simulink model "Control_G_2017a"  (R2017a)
settings: Solver=ode113  StartTime=0  StopTime=80  FixedStep=0.01  MaxStep=0.001  RelTol=1e-3  AbsTol=1e-5
undefined symbols (not defined in the file or in its folder): lower_limit, upper_limit, X0

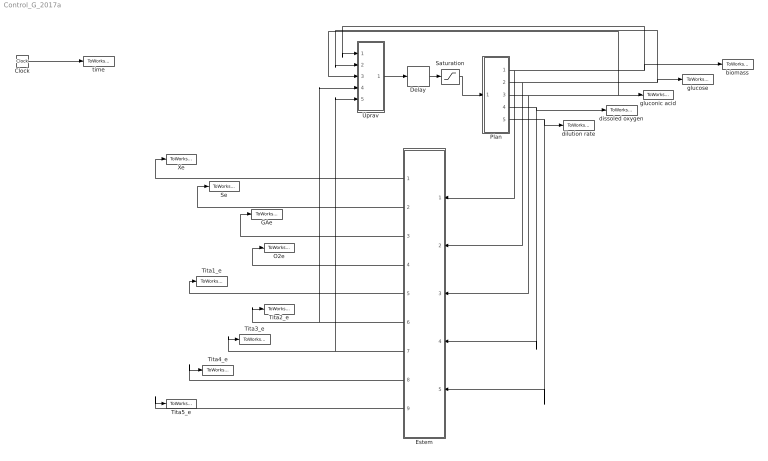
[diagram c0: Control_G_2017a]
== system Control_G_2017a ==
  Clock : Clock
  Delay : TransportDelay  DelayTime=0.0001
  Estem : Subsystem
  GAe : ToWorkspace  VariableName=GAe  SampleTime=0.1
  O2e : ToWorkspace  VariableName=O2e  SampleTime=0.1
  Plan : Subsystem
  Saturation : Saturate  UpperLimit=1  LowerLimit=0.0001
  Se : ToWorkspace  VariableName=Ge  SampleTime=0.1
  Tita1_e : ToWorkspace  VariableName=Tita1_e  SampleTime=0.1
  Tita2_e : ToWorkspace  VariableName=Tita2_e  SampleTime=0.1
  Tita3_e : ToWorkspace  VariableName=Tita3_e  SampleTime=0.1
  Tita4_e : ToWorkspace  VariableName=Tita4_e  SampleTime=0.1
  Tita5_e : ToWorkspace  VariableName=Tita5_e  SampleTime=0.1
  Uprav : Subsystem
  Xe : ToWorkspace  VariableName=Xe  SampleTime=0.1
  biomass : ToWorkspace  VariableName=Xm  SampleTime=0.1
  dilution rate : ToWorkspace  VariableName=D  SampleTime=0.1
  dissoled oxygen : ToWorkspace  VariableName=O2m  SampleTime=0.1
  gluconic acid : ToWorkspace  VariableName=GAm  SampleTime=0.1
  glucose : ToWorkspace  VariableName=Gm  SampleTime=0.1
  time : ToWorkspace  VariableName=time  SampleTime=0.1
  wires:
  Delay/1 -> Saturation/1
  Plan/1(X) -> Estem/1(X), Uprav/1(Xe), biomass/1
  Plan/2(S) -> Uprav/2(Se), glucose/1, Estem/2(S)
  Plan/3(GA) -> Uprav/3(GAe), gluconic acid/1, Estem/3(GA)
  Plan/5(D) -> Estem/5(Din), dilution rate/1
  Uprav/1(D_) -> Delay/1
  Saturation/1 -> Plan/1(D1)
  Plan/4(O2) -> Estem/4(O2), dissoled oxygen/1
  Estem/1(Xe) -> Xe/1
  Estem/2(Se) -> Se/1
  Estem/4(O2e) -> O2e/1
  Estem/5(Tita_1) -> Tita1_e/1
  Estem/7(Tita_3) -> Tita3_e/1, Uprav/5(tita_3)
  Estem/3(GAe) -> GAe/1
  Estem/8(Tita_4) -> Tita4_e/1
  Estem/9(Tita_5) -> Tita5_e/1
  Estem/6(Tita_2) -> Tita2_e/1, Uprav/4(tita_2)
  Clock/1 -> time/1

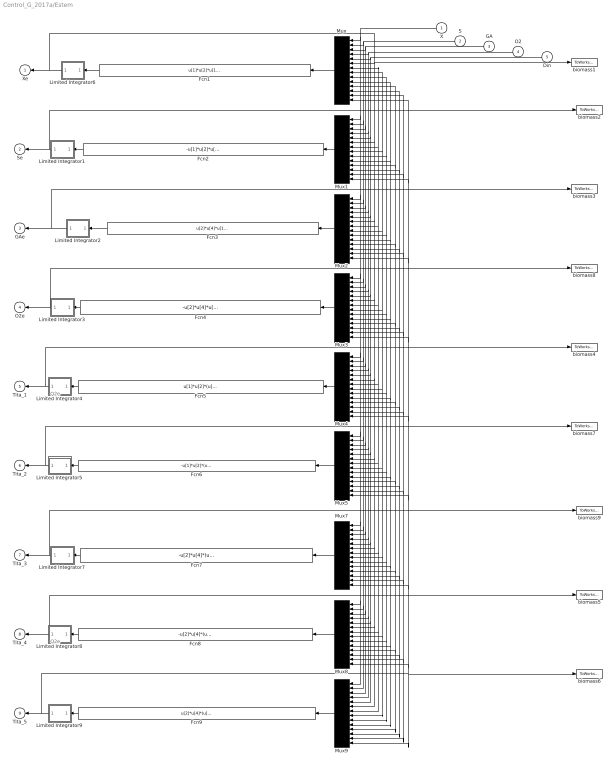
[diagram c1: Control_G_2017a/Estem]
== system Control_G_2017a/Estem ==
  note: Q2e
  note: Q2e
  X : Inport
  S : Inport  Port=2
  GA : Inport  Port=3
  O2 : Inport  Port=4
  Din : Inport  Port=5
  Fcn1 : Fcn  Expr=u[1]*u[2]*u[10]-u[5]*u[1]+1*(u[1]-u[6])
  Fcn2 : Fcn  Expr=-u[1]*u[2]*u[11]-u[2]*u[4]*u[12]-u[5]*(u[2]-200)+1*(u[2]-u[7])
  Fcn3 : Fcn  Expr=u[2]*u[4]*u[14]-u[5]*u[3]+1*(u[3]-u[8])
  Fcn4 : Fcn  Expr=-u[2]*u[4]*u[13]-u[5]*u[4]+600*(0.0075- u[4])+1*(u[4]-u[9])
  Fcn5 : Fcn  Expr=u[1]*u[2]*(u[1]-u[6])/(4*(u[1]*u[2]*u[1]*u[2]))
  Fcn6 : Fcn  Expr=-u[1]*u[2]*(u[2]-u[7])/(4*(u[1]*u[2]*u[1]*u[2]+u[2]*u[4]*u[2]*u[4]))
  Fcn7 : Fcn  Expr=-u[2]*u[4]*(u[2]-u[7])/(4*(u[1]*u[2]*u[1]*u[2]+u[2]*u[4]*u[2]*u[4]))
  Fcn8 : Fcn  Expr=-u[2]*u[4]*(u[4]-u[9])/(4*u[2]*u[4]*u[2]*u[4])
  Fcn9 : Fcn  Expr=u[2]*u[4]*(u[3]-u[8])/(4*u[2]*u[4]*u[2]*u[4])
  Limited Integrator1 : Subsystem
  Limited Integrator2 : Subsystem
  Limited Integrator3 : Subsystem
  Limited Integrator4 : Subsystem
  Limited Integrator5 : Subsystem
  Limited Integrator6 : Subsystem
  Limited Integrator7 : Subsystem
  Limited Integrator8 : Subsystem
  Limited Integrator9 : Subsystem
  Mux{,1..5,7..9} (9 alike) : Mux  Inputs=14
  biomass1 : ToWorkspace  VariableName=Xest  SampleTime=0.1
  biomass2 : ToWorkspace  VariableName=Sest  SampleTime=0.1
  biomass3 : ToWorkspace  VariableName=GAest  SampleTime=0.1
  biomass4 : ToWorkspace  VariableName=Tita1  SampleTime=0.1
  biomass5 : ToWorkspace  VariableName=Tita4  SampleTime=0.1
  biomass6 : ToWorkspace  VariableName=Tita5  SampleTime=0.1
  biomass7 : ToWorkspace  VariableName=Tita2  SampleTime=0.1
  biomass8 : ToWorkspace  VariableName=O2est  SampleTime=0.1
  biomass9 : ToWorkspace  VariableName=Tita3  SampleTime=0.1
  Xe : Outport  InitialOutput=0
  Se : Outport  Port=2  InitialOutput=0
  GAe : Outport  Port=3  InitialOutput=0
  O2e : Outport  Port=4  InitialOutput=0
  Tita_1 : Outport  Port=5  InitialOutput=0
  Tita_2 : Outport  Port=6  InitialOutput=0
  Tita_3 : Outport  Port=7  InitialOutput=0
  Tita_4 : Outport  Port=8  InitialOutput=0
  Tita_5 : Outport  Port=9  InitialOutput=0
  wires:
  Mux/1 -> Fcn1/1
  Fcn1/1 -> Limited Integrator6/1(Inport)
  Mux1/1 -> Fcn2/1
  Mux2/1 -> Fcn3/1
  Fcn3/1 -> Limited Integrator2/1(Inport)
  Fcn4/1 -> Limited Integrator3/1(Inport)
  Mux3/1 -> Fcn4/1
  Mux4/1 -> Fcn5/1
  Fcn5/1 -> Limited Integrator4/1(Inport)
  Fcn6/1 -> Limited Integrator5/1(Inport)
  Mux5/1 -> Fcn6/1
  X/1 -> Mux/1, Mux9/1, Mux8/1, Mux7/1, Mux5/1, Mux4/1, Mux3/1, Mux2/1, Mux1/1
  S/1 -> Mux9/2, Mux8/2, Mux7/2, Mux5/2, Mux4/2, Mux3/2, Mux2/2, Mux1/2, Mux/2
  GA/1 -> Mux1/3, Mux2/3, Mux3/3, Mux8/3, Mux9/3, Mux7/3, Mux5/3, Mux4/3, Mux/3
  O2/1 -> Mux1/4, Mux2/4, Mux3/4, Mux9/4, Mux8/4, Mux7/4, Mux5/4, Mux4/4, Mux/4
  Din/1 -> Mux1/5, Mux2/5, Mux3/5, Mux9/5, Mux8/5, Mux7/5, Mux5/5, Mux4/5, Mux/5
  Mux9/1 -> Fcn9/1
  Fcn9/1 -> Limited Integrator9/1(Inport)
  Mux7/1 -> Fcn7/1
  Fcn7/1 -> Limited Integrator7/1(Inport)
  Fcn8/1 -> Limited Integrator8/1(Inport)
  Mux8/1 -> Fcn8/1
  Fcn2/1 -> Limited Integrator1/1(Inport)
  Limited Integrator2/1(Outport) -> GAe/1, biomass3/1, Mux9/8, Mux8/8, Mux7/8, Mux5/8, Mux4/8, Mux3/8, Mux2/8, Mux1/8, Mux/8
  Limited Integrator1/1(Outport) -> Mux/7, Mux9/7, Mux8/7, Mux7/7, Mux5/7, Mux4/7, Mux3/7, Mux2/7, Mux1/7, biomass2/1, Se/1
  Limited Integrator3/1(Outport) -> biomass8/1, Mux9/9, Mux8/9, Mux7/9, Mux5/9, Mux4/9, Mux3/9, Mux2/9, Mux/9, Mux1/9, O2e/1
  Limited Integrator4/1(Outport) -> biomass4/1, Mux5/10, Mux9/10, Mux8/10, Mux7/10, Mux4/10, Mux3/10, Mux2/10, Mux1/10, Mux/10, Tita_1/1
  Limited Integrator5/1(Outport) -> biomass7/1, Mux/11, Mux1/11, Mux2/11, Mux3/11, Mux4/11, Mux9/11, Mux8/11, Mux7/11, Mux5/11, Tita_2/1
  Limited Integrator9/1(Outport) -> biomass6/1, Mux9/14, Mux/14, Mux1/14, Mux2/14, Mux3/14, Mux4/14, Mux5/14, Mux7/14, Mux8/14, Tita_5/1
  Limited Integrator6/1(Outport) -> Xe/1, Mux9/6, Mux8/6, Mux7/6, Mux5/6, Mux4/6, Mux3/6, Mux2/6, Mux1/6, biomass1/1, Mux/6
  Limited Integrator7/1(Outport) -> biomass9/1, Mux9/12, Mux8/12, Mux7/12, Mux/12, Mux1/12, Mux2/12, Mux3/12, Mux4/12, Mux5/12, Tita_3/1
  Limited Integrator8/1(Outport) -> biomass5/1, Mux9/13, Mux8/13, Mux/13, Mux1/13, Mux2/13, Mux3/13, Mux4/13, Mux5/13, Mux7/13, Tita_4/1

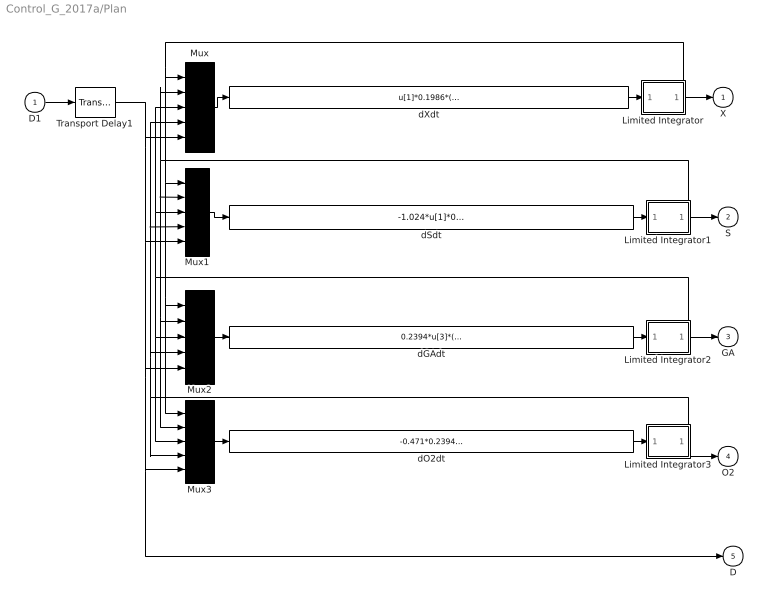
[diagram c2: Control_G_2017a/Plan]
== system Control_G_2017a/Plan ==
  D1 : Inport
  Limited Integrator : Subsystem
  Limited Integrator1 : Subsystem
  Limited Integrator2 : Subsystem
  Limited Integrator3 : Subsystem
  Mux{,1..3} (4 alike) : Mux  Inputs=5
  Transport Delay1 : TransportDelay  DelayTime=0.0001  BufferSize=100024
  dGAdt : Fcn  Expr=0.2394*u[3]*(146.0696-u[3])/146.0696-u[5]*u[3]
  dO2dt : Fcn  Expr=-0.471*0.2394*u[3]*(146.0696-u[3])/146.0696+600*(0.0075-u[4])-u[5]*u[4]
  dSdt : Fcn  Expr=-1.024*u[1]*0.1986*(3.1114-u[1])/3.1114-1.1647*0.2394*u[3]*(146.0696-u[3])/146.0696-u[5]*(u[2]-200)
  dXdt : Fcn  Expr=u[1]*0.1986*(3.1114-u[1])/3.1114-u[5]*u[1]
  X : Outport  InitialOutput=0
  S : Outport  Port=2  InitialOutput=0
  GA : Outport  Port=3  InitialOutput=0
  O2 : Outport  Port=4  InitialOutput=0
  D : Outport  Port=5  InitialOutput=0
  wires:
  Mux/1 -> dXdt/1
  dXdt/1 -> Limited Integrator/1(Inport)
  dSdt/1 -> Limited Integrator1/1(Inport)
  dGAdt/1 -> Limited Integrator2/1(Inport)
  dO2dt/1 -> Limited Integrator3/1(Inport)
  Mux1/1 -> dSdt/1
  Mux2/1 -> dGAdt/1
  Limited Integrator/1(Outport) -> X/1, Mux3/1, Mux2/1, Mux1/1, Mux/1
  Limited Integrator1/1(Outport) -> S/1, Mux/2, Mux1/2, Mux3/2, Mux2/2
  Limited Integrator2/1(Outport) -> GA/1, Mux2/3, Mux3/3, Mux1/3, Mux/3
  Limited Integrator3/1(Outport) -> O2/1, Mux3/4, Mux2/4, Mux1/4, Mux/4
  D1/1 -> Transport Delay1/1
  Mux3/1 -> dO2dt/1
  Transport Delay1/1 -> D/1, Mux3/5, Mux2/5, Mux1/5, Mux/5

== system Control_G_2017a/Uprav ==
  Xe : Inport
  Se : Inport  Port=2
  GAe : Inport  Port=3
  tita_2 : Inport  Port=4
  tita_3 : Inport  Port=5
  FcnU : Fcn  Expr=(-15*(3-u[2])-u[1]*u[2]*u[4]-u[2]*u[3]*u[5])/(u[2]-200)
  Mux : Mux  Inputs=5
  D_ : Outport  InitialOutput=0
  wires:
  FcnU/1 -> D_/1
  tita_2/1 -> Mux/4
  GAe/1 -> Mux/3
  Se/1 -> Mux/2
  Xe/1 -> Mux/1
  Mux/1 -> FcnU/1
  tita_3/1 -> Mux/5

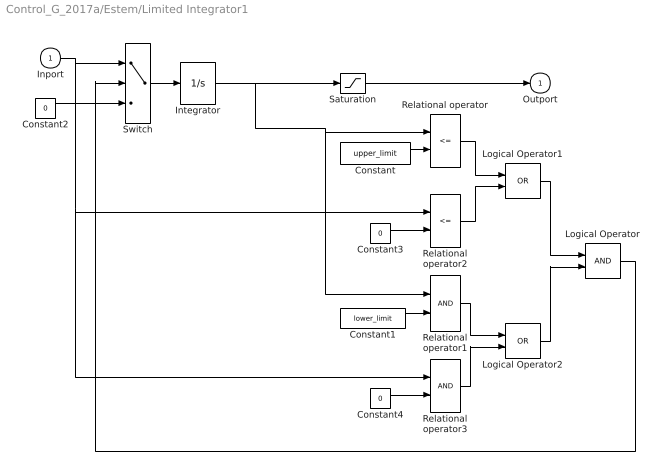
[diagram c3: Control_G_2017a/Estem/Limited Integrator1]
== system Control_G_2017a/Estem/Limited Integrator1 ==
  Inport : Inport
  Constant : Constant  Value=upper_limit
  Constant1 : Constant  Value=lower_limit
  Constant2 : Constant  Value=0
  Constant3 : Constant  Value=0
  Constant4 : Constant  Value=0
  Integrator : Integrator  InitialCondition=X0
  Logical Operator : Logic
  Logical Operator1 : Logic  Operator=OR
  Logical Operator2 : Logic  Operator=OR
  Relational operator : RelationalOperator  Operator=<=
  Relational operator1 : RelationalOperator
  Relational operator2 : RelationalOperator  Operator=<=
  Relational operator3 : RelationalOperator
  Saturation : Saturate  UpperLimit=upper_limit  LowerLimit=lower_limit
  Switch : Switch  Threshold=0.5
  Outport : Outport  InitialOutput=0
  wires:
  Saturation/1 -> Outport/1
  Inport/1 -> Switch/1, Relational operator2/1, Relational operator3/1
  Switch/1 -> Integrator/1
  Constant/1 -> Relational operator/2
  Constant1/1 -> Relational operator1/2
  Logical Operator/1 -> Switch/2
  Constant2/1 -> Switch/3
  Relational operator/1 -> Logical Operator1/1
  Relational operator2/1 -> Logical Operator1/2
  Logical Operator1/1 -> Logical Operator/1
  Relational operator1/1 -> Logical Operator2/1
  Relational operator3/1 -> Logical Operator2/2
  Logical Operator2/1 -> Logical Operator/2
  Constant3/1 -> Relational operator2/2
  Constant4/1 -> Relational operator3/2
  Integrator/1 -> Saturation/1, Relational operator1/1, Relational operator/1

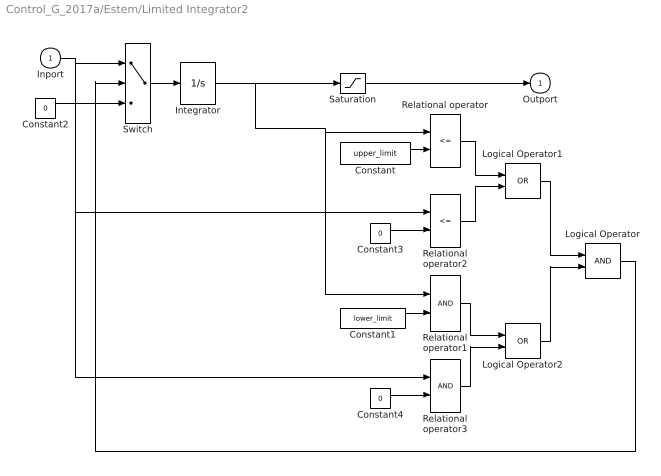
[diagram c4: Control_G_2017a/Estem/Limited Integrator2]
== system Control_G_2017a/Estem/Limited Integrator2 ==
  Inport : Inport
  Constant : Constant  Value=upper_limit
  Constant1 : Constant  Value=lower_limit
  Constant2 : Constant  Value=0
  Constant3 : Constant  Value=0
  Constant4 : Constant  Value=0
  Integrator : Integrator  InitialCondition=X0
  Logical Operator : Logic
  Logical Operator1 : Logic  Operator=OR
  Logical Operator2 : Logic  Operator=OR
  Relational operator : RelationalOperator  Operator=<=
  Relational operator1 : RelationalOperator
  Relational operator2 : RelationalOperator  Operator=<=
  Relational operator3 : RelationalOperator
  Saturation : Saturate  UpperLimit=upper_limit  LowerLimit=lower_limit
  Switch : Switch  Threshold=0.5
  Outport : Outport  InitialOutput=0
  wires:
  Constant4/1 -> Relational operator3/2
  Constant3/1 -> Relational operator2/2
  Logical Operator2/1 -> Logical Operator/2
  Relational operator3/1 -> Logical Operator2/2
  Relational operator1/1 -> Logical Operator2/1
  Logical Operator1/1 -> Logical Operator/1
  Relational operator2/1 -> Logical Operator1/2
  Relational operator/1 -> Logical Operator1/1
  Constant2/1 -> Switch/3
  Logical Operator/1 -> Switch/2
  Constant1/1 -> Relational operator1/2
  Constant/1 -> Relational operator/2
  Switch/1 -> Integrator/1
  Inport/1 -> Switch/1, Relational operator2/1, Relational operator3/1
  Integrator/1 -> Relational operator1/1, Relational operator/1, Saturation/1
  Saturation/1 -> Outport/1

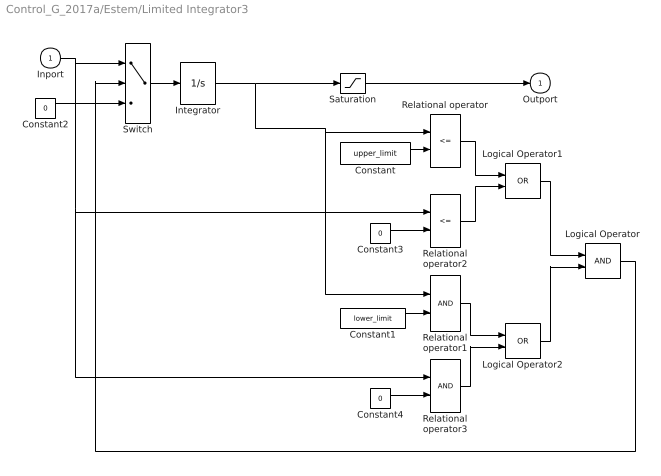
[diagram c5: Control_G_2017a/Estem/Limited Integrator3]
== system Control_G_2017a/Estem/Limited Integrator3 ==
  Inport : Inport
  Constant : Constant  Value=upper_limit
  Constant1 : Constant  Value=lower_limit
  Constant2 : Constant  Value=0
  Constant3 : Constant  Value=0
  Constant4 : Constant  Value=0
  Integrator : Integrator  InitialCondition=X0
  Logical Operator : Logic
  Logical Operator1 : Logic  Operator=OR
  Logical Operator2 : Logic  Operator=OR
  Relational operator : RelationalOperator  Operator=<=
  Relational operator1 : RelationalOperator
  Relational operator2 : RelationalOperator  Operator=<=
  Relational operator3 : RelationalOperator
  Saturation : Saturate  UpperLimit=upper_limit  LowerLimit=lower_limit
  Switch : Switch  Threshold=0.5
  Outport : Outport  InitialOutput=0
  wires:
  Saturation/1 -> Outport/1
  Inport/1 -> Switch/1, Relational operator2/1, Relational operator3/1
  Switch/1 -> Integrator/1
  Constant/1 -> Relational operator/2
  Constant1/1 -> Relational operator1/2
  Logical Operator/1 -> Switch/2
  Constant2/1 -> Switch/3
  Relational operator/1 -> Logical Operator1/1
  Relational operator2/1 -> Logical Operator1/2
  Logical Operator1/1 -> Logical Operator/1
  Relational operator1/1 -> Logical Operator2/1
  Relational operator3/1 -> Logical Operator2/2
  Logical Operator2/1 -> Logical Operator/2
  Constant3/1 -> Relational operator2/2
  Constant4/1 -> Relational operator3/2
  Integrator/1 -> Saturation/1, Relational operator1/1, Relational operator/1

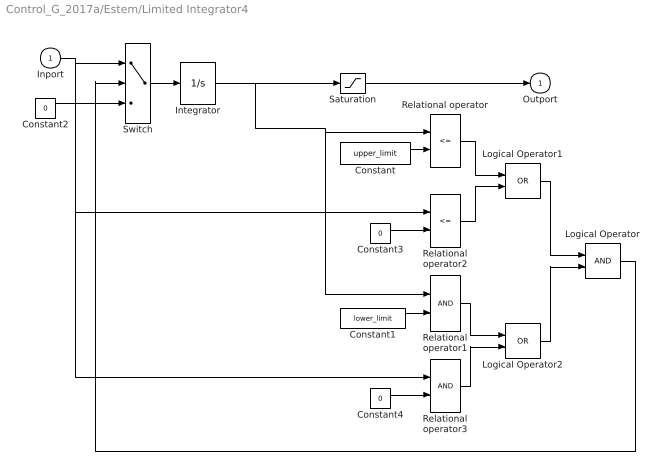
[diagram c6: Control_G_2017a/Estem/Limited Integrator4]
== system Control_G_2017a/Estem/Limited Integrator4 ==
  Inport : Inport
  Constant : Constant  Value=upper_limit
  Constant1 : Constant  Value=lower_limit
  Constant2 : Constant  Value=0
  Constant3 : Constant  Value=0
  Constant4 : Constant  Value=0
  Integrator : Integrator  InitialCondition=X0
  Logical Operator : Logic
  Logical Operator1 : Logic  Operator=OR
  Logical Operator2 : Logic  Operator=OR
  Relational operator : RelationalOperator  Operator=<=
  Relational operator1 : RelationalOperator
  Relational operator2 : RelationalOperator  Operator=<=
  Relational operator3 : RelationalOperator
  Saturation : Saturate  UpperLimit=upper_limit  LowerLimit=lower_limit
  Switch : Switch  Threshold=0.5
  Outport : Outport  InitialOutput=0
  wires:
  Constant4/1 -> Relational operator3/2
  Constant3/1 -> Relational operator2/2
  Logical Operator2/1 -> Logical Operator/2
  Relational operator3/1 -> Logical Operator2/2
  Relational operator1/1 -> Logical Operator2/1
  Logical Operator1/1 -> Logical Operator/1
  Relational operator2/1 -> Logical Operator1/2
  Relational operator/1 -> Logical Operator1/1
  Constant2/1 -> Switch/3
  Logical Operator/1 -> Switch/2
  Constant1/1 -> Relational operator1/2
  Constant/1 -> Relational operator/2
  Switch/1 -> Integrator/1
  Inport/1 -> Switch/1, Relational operator2/1, Relational operator3/1
  Integrator/1 -> Relational operator1/1, Relational operator/1, Saturation/1
  Saturation/1 -> Outport/1

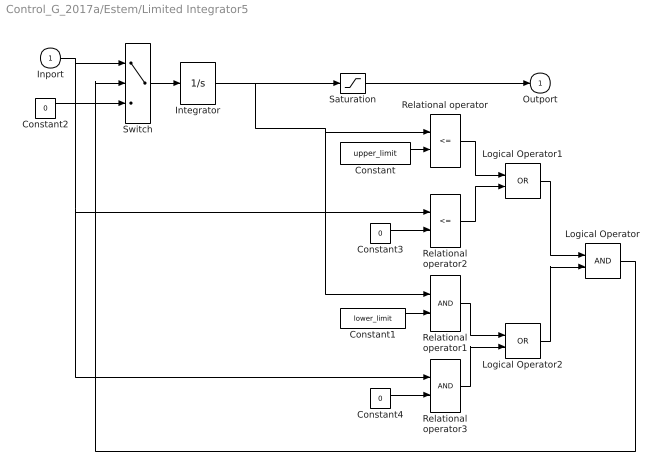
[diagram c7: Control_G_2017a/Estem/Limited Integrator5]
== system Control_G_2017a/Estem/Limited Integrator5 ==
  Inport : Inport
  Constant : Constant  Value=upper_limit
  Constant1 : Constant  Value=lower_limit
  Constant2 : Constant  Value=0
  Constant3 : Constant  Value=0
  Constant4 : Constant  Value=0
  Integrator : Integrator  InitialCondition=X0
  Logical Operator : Logic
  Logical Operator1 : Logic  Operator=OR
  Logical Operator2 : Logic  Operator=OR
  Relational operator : RelationalOperator  Operator=<=
  Relational operator1 : RelationalOperator
  Relational operator2 : RelationalOperator  Operator=<=
  Relational operator3 : RelationalOperator
  Saturation : Saturate  UpperLimit=upper_limit  LowerLimit=lower_limit
  Switch : Switch  Threshold=0.5
  Outport : Outport  InitialOutput=0
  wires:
  Saturation/1 -> Outport/1
  Inport/1 -> Switch/1, Relational operator2/1, Relational operator3/1
  Switch/1 -> Integrator/1
  Constant/1 -> Relational operator/2
  Constant1/1 -> Relational operator1/2
  Logical Operator/1 -> Switch/2
  Constant2/1 -> Switch/3
  Relational operator/1 -> Logical Operator1/1
  Relational operator2/1 -> Logical Operator1/2
  Logical Operator1/1 -> Logical Operator/1
  Relational operator1/1 -> Logical Operator2/1
  Relational operator3/1 -> Logical Operator2/2
  Logical Operator2/1 -> Logical Operator/2
  Constant3/1 -> Relational operator2/2
  Constant4/1 -> Relational operator3/2
  Integrator/1 -> Saturation/1, Relational operator1/1, Relational operator/1

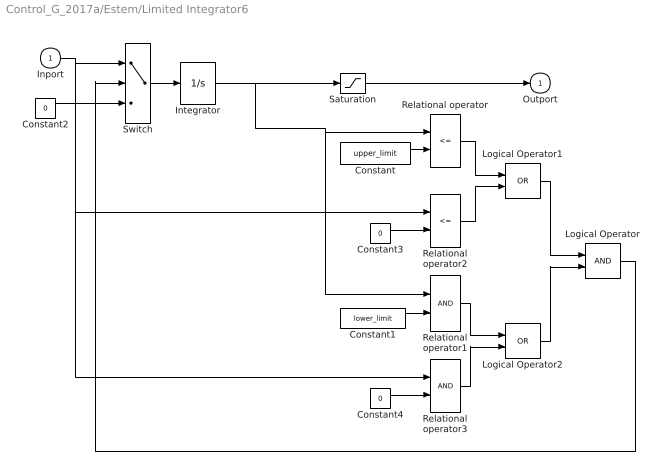
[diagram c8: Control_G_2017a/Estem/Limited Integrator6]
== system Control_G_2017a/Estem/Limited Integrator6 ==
  Inport : Inport
  Constant : Constant  Value=upper_limit
  Constant1 : Constant  Value=lower_limit
  Constant2 : Constant  Value=0
  Constant3 : Constant  Value=0
  Constant4 : Constant  Value=0
  Integrator : Integrator  InitialCondition=X0
  Logical Operator : Logic
  Logical Operator1 : Logic  Operator=OR
  Logical Operator2 : Logic  Operator=OR
  Relational operator : RelationalOperator  Operator=<=
  Relational operator1 : RelationalOperator
  Relational operator2 : RelationalOperator  Operator=<=
  Relational operator3 : RelationalOperator
  Saturation : Saturate  UpperLimit=upper_limit  LowerLimit=lower_limit
  Switch : Switch  Threshold=0.5
  Outport : Outport  InitialOutput=0
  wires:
  Constant4/1 -> Relational operator3/2
  Constant3/1 -> Relational operator2/2
  Logical Operator2/1 -> Logical Operator/2
  Relational operator3/1 -> Logical Operator2/2
  Relational operator1/1 -> Logical Operator2/1
  Logical Operator1/1 -> Logical Operator/1
  Relational operator2/1 -> Logical Operator1/2
  Relational operator/1 -> Logical Operator1/1
  Constant2/1 -> Switch/3
  Logical Operator/1 -> Switch/2
  Constant1/1 -> Relational operator1/2
  Constant/1 -> Relational operator/2
  Switch/1 -> Integrator/1
  Inport/1 -> Switch/1, Relational operator2/1, Relational operator3/1
  Integrator/1 -> Relational operator1/1, Relational operator/1, Saturation/1
  Saturation/1 -> Outport/1

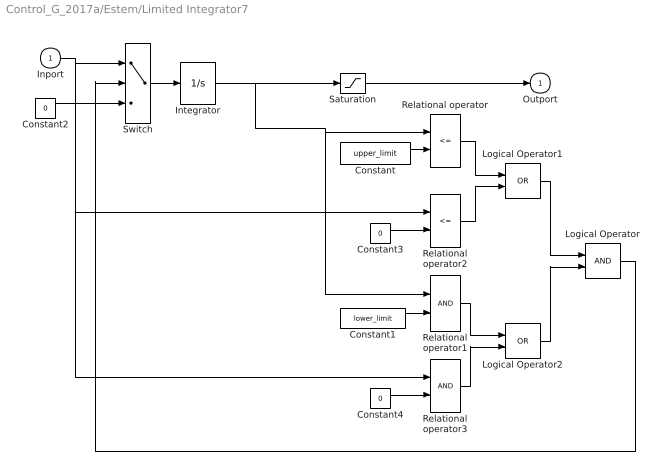
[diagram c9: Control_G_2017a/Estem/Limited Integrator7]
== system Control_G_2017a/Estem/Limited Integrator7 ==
  Inport : Inport
  Constant : Constant  Value=upper_limit
  Constant1 : Constant  Value=lower_limit
  Constant2 : Constant  Value=0
  Constant3 : Constant  Value=0
  Constant4 : Constant  Value=0
  Integrator : Integrator  InitialCondition=X0
  Logical Operator : Logic
  Logical Operator1 : Logic  Operator=OR
  Logical Operator2 : Logic  Operator=OR
  Relational operator : RelationalOperator  Operator=<=
  Relational operator1 : RelationalOperator
  Relational operator2 : RelationalOperator  Operator=<=
  Relational operator3 : RelationalOperator
  Saturation : Saturate  UpperLimit=upper_limit  LowerLimit=lower_limit
  Switch : Switch  Threshold=0.5
  Outport : Outport  InitialOutput=0
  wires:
  Saturation/1 -> Outport/1
  Inport/1 -> Switch/1, Relational operator2/1, Relational operator3/1
  Switch/1 -> Integrator/1
  Constant/1 -> Relational operator/2
  Constant1/1 -> Relational operator1/2
  Logical Operator/1 -> Switch/2
  Constant2/1 -> Switch/3
  Relational operator/1 -> Logical Operator1/1
  Relational operator2/1 -> Logical Operator1/2
  Logical Operator1/1 -> Logical Operator/1
  Relational operator1/1 -> Logical Operator2/1
  Relational operator3/1 -> Logical Operator2/2
  Logical Operator2/1 -> Logical Operator/2
  Constant3/1 -> Relational operator2/2
  Constant4/1 -> Relational operator3/2
  Integrator/1 -> Saturation/1, Relational operator1/1, Relational operator/1

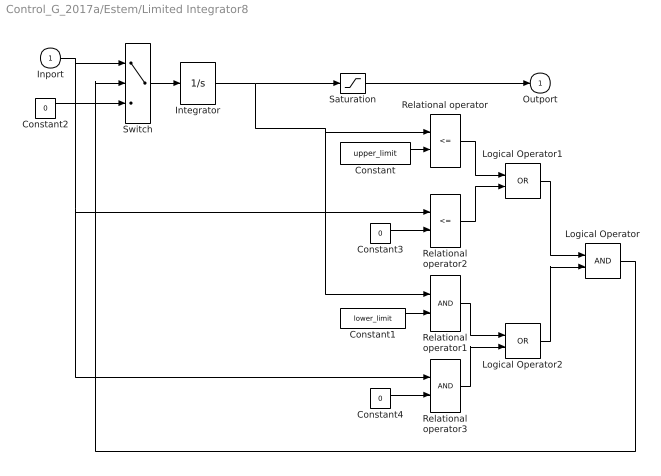
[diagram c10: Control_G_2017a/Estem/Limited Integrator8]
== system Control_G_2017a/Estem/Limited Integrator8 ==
  Inport : Inport
  Constant : Constant  Value=upper_limit
  Constant1 : Constant  Value=lower_limit
  Constant2 : Constant  Value=0
  Constant3 : Constant  Value=0
  Constant4 : Constant  Value=0
  Integrator : Integrator  InitialCondition=X0
  Logical Operator : Logic
  Logical Operator1 : Logic  Operator=OR
  Logical Operator2 : Logic  Operator=OR
  Relational operator : RelationalOperator  Operator=<=
  Relational operator1 : RelationalOperator
  Relational operator2 : RelationalOperator  Operator=<=
  Relational operator3 : RelationalOperator
  Saturation : Saturate  UpperLimit=upper_limit  LowerLimit=lower_limit
  Switch : Switch  Threshold=0.5
  Outport : Outport  InitialOutput=0
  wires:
  Constant4/1 -> Relational operator3/2
  Constant3/1 -> Relational operator2/2
  Logical Operator2/1 -> Logical Operator/2
  Relational operator3/1 -> Logical Operator2/2
  Relational operator1/1 -> Logical Operator2/1
  Logical Operator1/1 -> Logical Operator/1
  Relational operator2/1 -> Logical Operator1/2
  Relational operator/1 -> Logical Operator1/1
  Constant2/1 -> Switch/3
  Logical Operator/1 -> Switch/2
  Constant1/1 -> Relational operator1/2
  Constant/1 -> Relational operator/2
  Switch/1 -> Integrator/1
  Inport/1 -> Switch/1, Relational operator2/1, Relational operator3/1
  Integrator/1 -> Relational operator1/1, Relational operator/1, Saturation/1
  Saturation/1 -> Outport/1

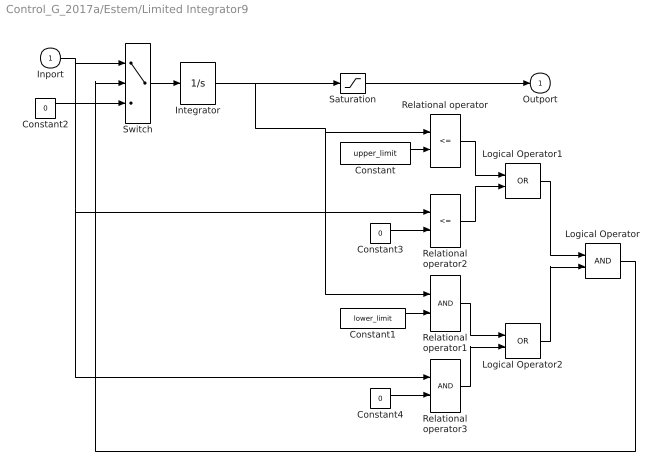
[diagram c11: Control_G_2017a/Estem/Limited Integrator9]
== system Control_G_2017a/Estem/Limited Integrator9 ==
  Inport : Inport
  Constant : Constant  Value=upper_limit
  Constant1 : Constant  Value=lower_limit
  Constant2 : Constant  Value=0
  Constant3 : Constant  Value=0
  Constant4 : Constant  Value=0
  Integrator : Integrator  InitialCondition=X0
  Logical Operator : Logic
  Logical Operator1 : Logic  Operator=OR
  Logical Operator2 : Logic  Operator=OR
  Relational operator : RelationalOperator  Operator=<=
  Relational operator1 : RelationalOperator
  Relational operator2 : RelationalOperator  Operator=<=
  Relational operator3 : RelationalOperator
  Saturation : Saturate  UpperLimit=upper_limit  LowerLimit=lower_limit
  Switch : Switch  Threshold=0.5
  Outport : Outport  InitialOutput=0
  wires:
  Saturation/1 -> Outport/1
  Inport/1 -> Switch/1, Relational operator2/1, Relational operator3/1
  Switch/1 -> Integrator/1
  Constant/1 -> Relational operator/2
  Constant1/1 -> Relational operator1/2
  Logical Operator/1 -> Switch/2
  Constant2/1 -> Switch/3
  Relational operator/1 -> Logical Operator1/1
  Relational operator2/1 -> Logical Operator1/2
  Logical Operator1/1 -> Logical Operator/1
  Relational operator1/1 -> Logical Operator2/1
  Relational operator3/1 -> Logical Operator2/2
  Logical Operator2/1 -> Logical Operator/2
  Constant3/1 -> Relational operator2/2
  Constant4/1 -> Relational operator3/2
  Integrator/1 -> Saturation/1, Relational operator1/1, Relational operator/1

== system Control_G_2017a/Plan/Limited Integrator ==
  Inport : Inport
  Constant : Constant  Value=upper_limit
  Constant1 : Constant  Value=lower_limit
  Constant2 : Constant  Value=0
  Constant3 : Constant  Value=0
  Constant4 : Constant  Value=0
  Integrator : Integrator  InitialCondition=0.01
  Logical Operator : Logic
  Logical Operator1 : Logic  Operator=OR
  Logical Operator2 : Logic  Operator=OR
  Relational operator : RelationalOperator  Operator=<=
  Relational operator1 : RelationalOperator
  Relational operator2 : RelationalOperator  Operator=<=
  Relational operator3 : RelationalOperator
  Saturation : Saturate  UpperLimit=upper_limit  LowerLimit=lower_limit
  Switch : Switch  Threshold=0.5
  Outport : Outport  InitialOutput=0
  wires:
  Constant4/1 -> Relational operator3/2
  Constant3/1 -> Relational operator2/2
  Logical Operator2/1 -> Logical Operator/2
  Relational operator3/1 -> Logical Operator2/2
  Relational operator1/1 -> Logical Operator2/1
  Logical Operator1/1 -> Logical Operator/1
  Relational operator2/1 -> Logical Operator1/2
  Relational operator/1 -> Logical Operator1/1
  Constant2/1 -> Switch/3
  Logical Operator/1 -> Switch/2
  Constant1/1 -> Relational operator1/2
  Constant/1 -> Relational operator/2
  Switch/1 -> Integrator/1
  Inport/1 -> Switch/1, Relational operator2/1, Relational operator3/1
  Integrator/1 -> Relational operator1/1, Relational operator/1, Saturation/1
  Saturation/1 -> Outport/1

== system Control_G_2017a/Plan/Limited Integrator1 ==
  Inport : Inport
  Constant : Constant  Value=upper_limit
  Constant1 : Constant  Value=lower_limit
  Constant2 : Constant  Value=0
  Constant3 : Constant  Value=0
  Constant4 : Constant  Value=0
  Integrator : Integrator  InitialCondition=X0
  Logical Operator : Logic
  Logical Operator1 : Logic  Operator=OR
  Logical Operator2 : Logic  Operator=OR
  Relational operator : RelationalOperator  Operator=<=
  Relational operator1 : RelationalOperator
  Relational operator2 : RelationalOperator  Operator=<=
  Relational operator3 : RelationalOperator
  Saturation : Saturate  UpperLimit=upper_limit  LowerLimit=lower_limit
  Switch : Switch  Threshold=0.5
  Outport : Outport  InitialOutput=0
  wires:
  Saturation/1 -> Outport/1
  Inport/1 -> Switch/1, Relational operator2/1, Relational operator3/1
  Switch/1 -> Integrator/1
  Constant/1 -> Relational operator/2
  Constant1/1 -> Relational operator1/2
  Logical Operator/1 -> Switch/2
  Constant2/1 -> Switch/3
  Relational operator/1 -> Logical Operator1/1
  Relational operator2/1 -> Logical Operator1/2
  Logical Operator1/1 -> Logical Operator/1
  Relational operator1/1 -> Logical Operator2/1
  Relational operator3/1 -> Logical Operator2/2
  Logical Operator2/1 -> Logical Operator/2
  Constant3/1 -> Relational operator2/2
  Constant4/1 -> Relational operator3/2
  Integrator/1 -> Saturation/1, Relational operator1/1, Relational operator/1

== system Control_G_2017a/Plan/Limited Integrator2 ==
  Inport : Inport
  Constant : Constant  Value=upper_limit
  Constant1 : Constant  Value=lower_limit
  Constant2 : Constant  Value=0
  Constant3 : Constant  Value=0
  Constant4 : Constant  Value=0
  Integrator : Integrator  InitialCondition=X0
  Logical Operator : Logic
  Logical Operator1 : Logic  Operator=OR
  Logical Operator2 : Logic  Operator=OR
  Relational operator : RelationalOperator  Operator=<=
  Relational operator1 : RelationalOperator
  Relational operator2 : RelationalOperator  Operator=<=
  Relational operator3 : RelationalOperator
  Saturation : Saturate  UpperLimit=upper_limit  LowerLimit=lower_limit
  Switch : Switch  Threshold=0.5
  Outport : Outport  InitialOutput=0
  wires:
  Constant4/1 -> Relational operator3/2
  Constant3/1 -> Relational operator2/2
  Logical Operator2/1 -> Logical Operator/2
  Relational operator3/1 -> Logical Operator2/2
  Relational operator1/1 -> Logical Operator2/1
  Logical Operator1/1 -> Logical Operator/1
  Relational operator2/1 -> Logical Operator1/2
  Relational operator/1 -> Logical Operator1/1
  Constant2/1 -> Switch/3
  Logical Operator/1 -> Switch/2
  Constant1/1 -> Relational operator1/2
  Constant/1 -> Relational operator/2
  Switch/1 -> Integrator/1
  Inport/1 -> Switch/1, Relational operator2/1, Relational operator3/1
  Integrator/1 -> Relational operator1/1, Relational operator/1, Saturation/1
  Saturation/1 -> Outport/1

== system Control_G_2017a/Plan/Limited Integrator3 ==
  Inport : Inport
  Constant : Constant  Value=upper_limit
  Constant1 : Constant  Value=lower_limit
  Constant2 : Constant  Value=0
  Constant3 : Constant  Value=0
  Constant4 : Constant  Value=0
  Integrator : Integrator  InitialCondition=X0
  Logical Operator : Logic
  Logical Operator1 : Logic  Operator=OR
  Logical Operator2 : Logic  Operator=OR
  Relational operator : RelationalOperator  Operator=<=
  Relational operator1 : RelationalOperator
  Relational operator2 : RelationalOperator  Operator=<=
  Relational operator3 : RelationalOperator
  Saturation : Saturate  UpperLimit=upper_limit  LowerLimit=lower_limit
  Switch : Switch  Threshold=0.5
  Outport : Outport  InitialOutput=0
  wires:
  Saturation/1 -> Outport/1
  Inport/1 -> Switch/1, Relational operator2/1, Relational operator3/1
  Switch/1 -> Integrator/1
  Constant/1 -> Relational operator/2
  Constant1/1 -> Relational operator1/2
  Logical Operator/1 -> Switch/2
  Constant2/1 -> Switch/3
  Relational operator/1 -> Logical Operator1/1
  Relational operator2/1 -> Logical Operator1/2
  Logical Operator1/1 -> Logical Operator/1
  Relational operator1/1 -> Logical Operator2/1
  Relational operator3/1 -> Logical Operator2/2
  Logical Operator2/1 -> Logical Operator/2
  Constant3/1 -> Relational operator2/2
  Constant4/1 -> Relational operator3/2
  Integrator/1 -> Saturation/1, Relational operator1/1, Relational operator/1
